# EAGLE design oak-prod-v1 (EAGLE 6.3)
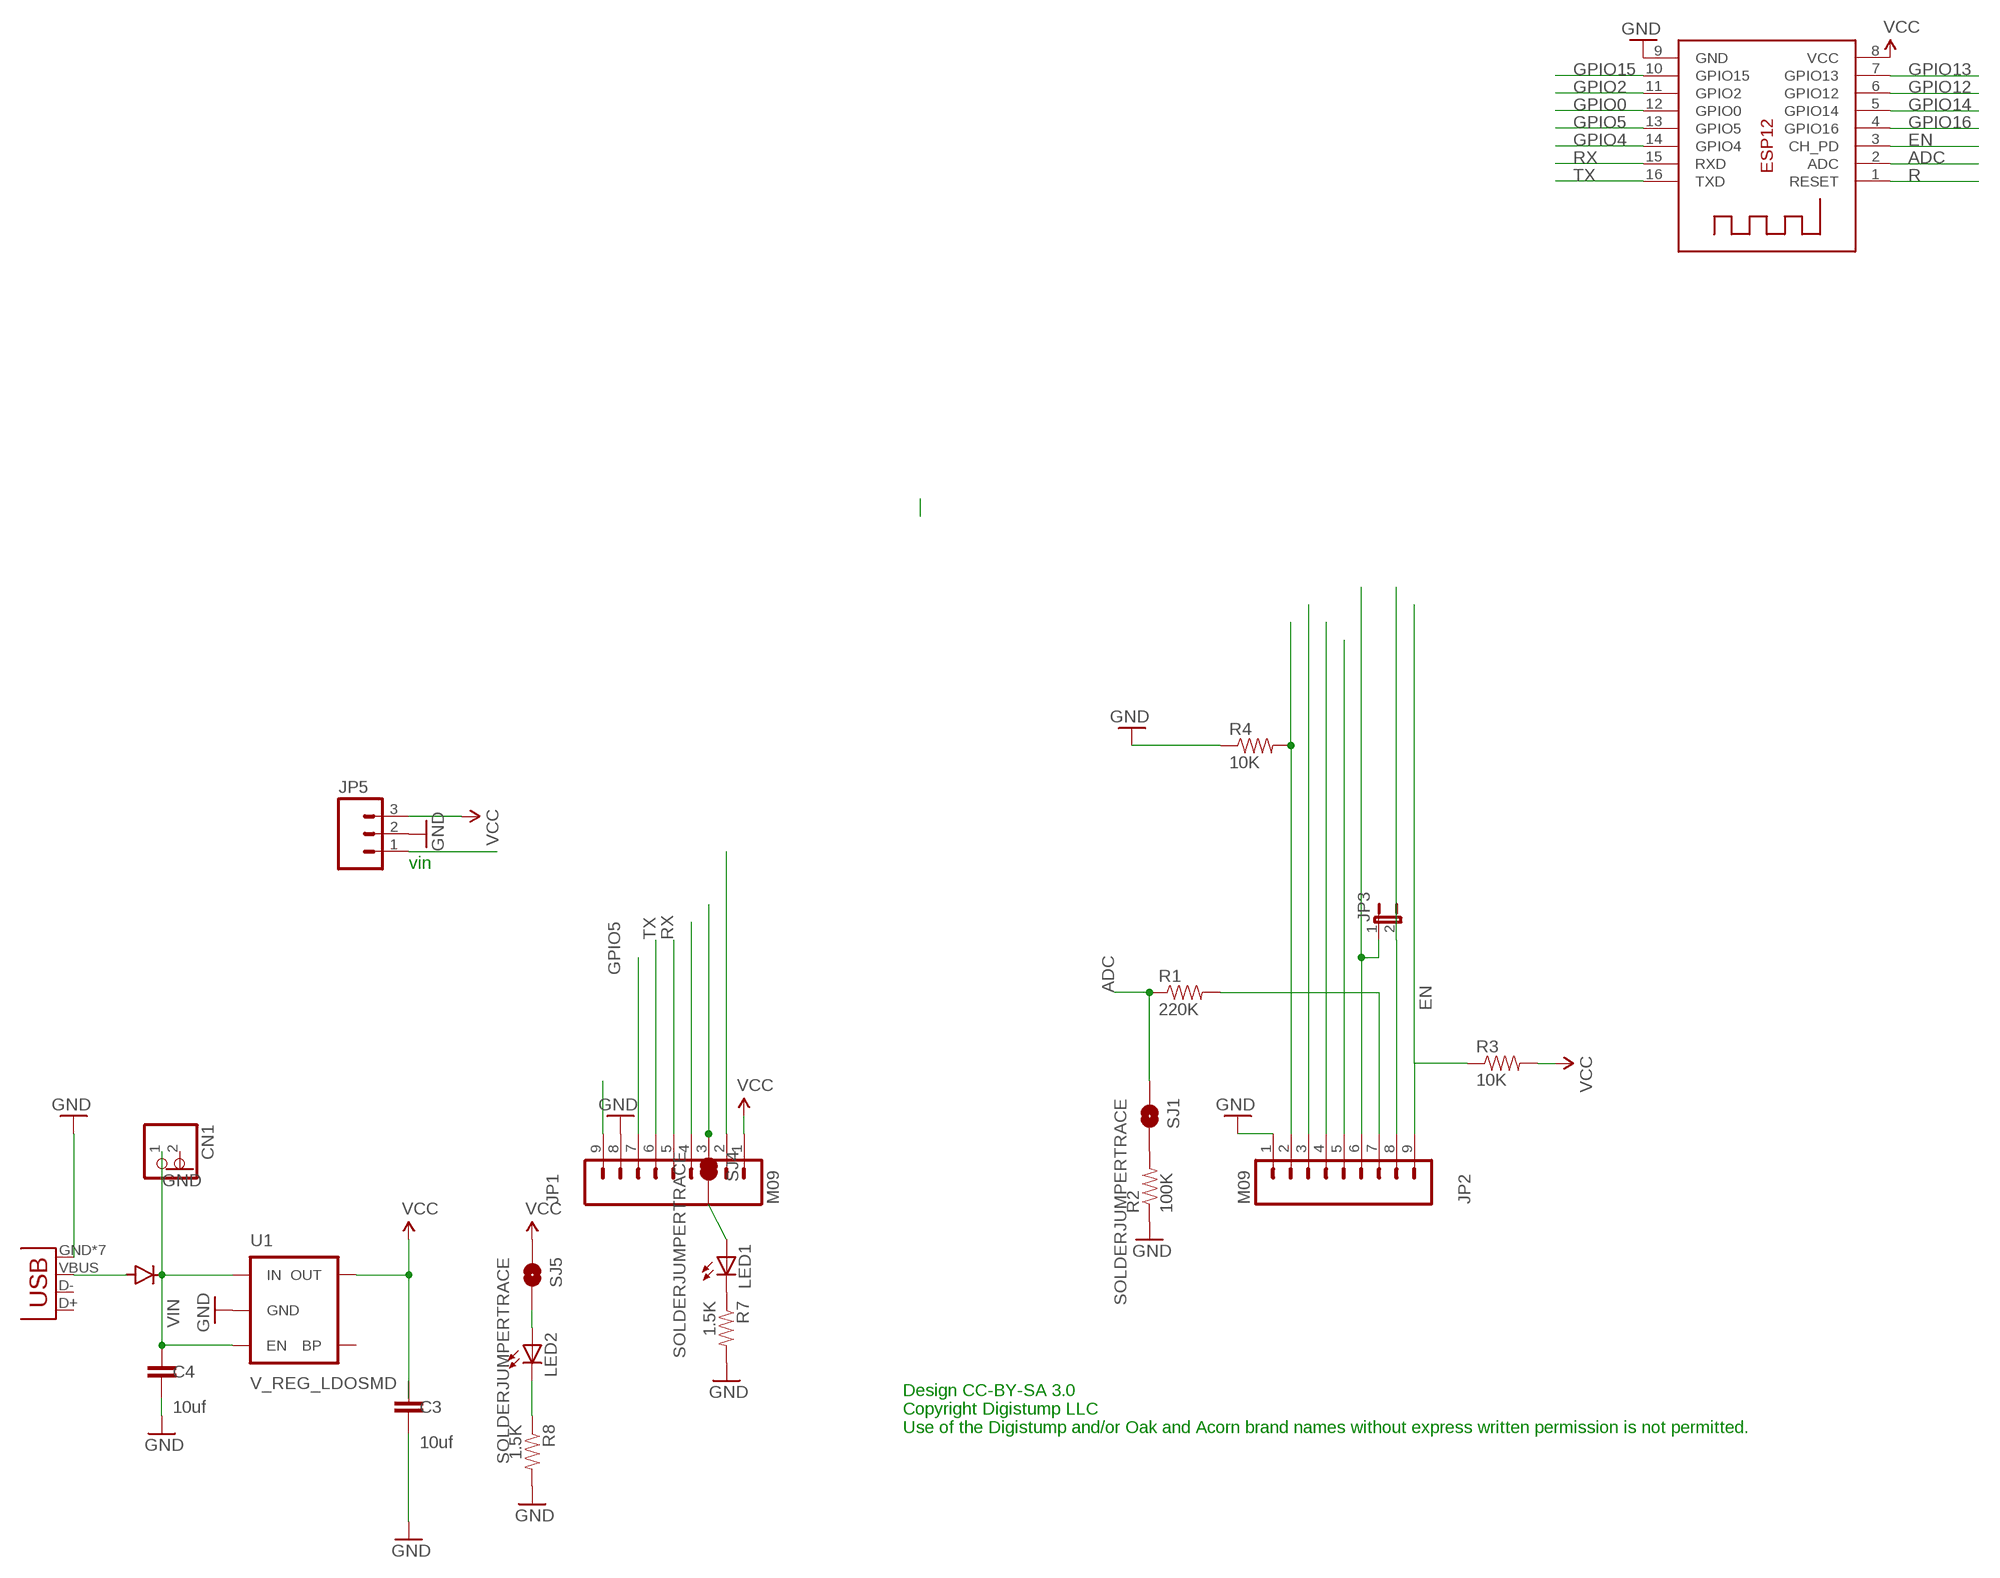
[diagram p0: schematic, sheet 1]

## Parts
C3  10uf  CAP0805  [0805]
C4  10uf  CAP0805  [0805]
CN1  JST_2PIN-THM-RA  [JST-PH-2-THM-RA]
D2  DIODE  [DIODE-DO-220AA(SMP)]
JP1  M09  [1X09]
JP2  M09  [1X09]
JP3  JUMPER-2SMD-NO  [SJ_2S-NO]
JP5  M03PTH  [1X03]
LED1  LEDCHIP-LED0805  [CHIP-LED0805]
LED2  LEDCHIP-LED0805  [CHIP-LED0805]
R1  220K  RESISTOR0603-RES  [0603-RES]
R2  100K  RESISTOR0603-RES  [0603-RES]
R3  10K  RESISTOR0603-RES  [0603-RES]
R4  10K  RESISTOR0603-RES  [0603-RES]
R7  1.5K  RESISTOR0603-RES  [0603-RES]
R8  1.5K  RESISTOR0603-RES  [0603-RES]
SJ1  SOLDERJUMPERTRACE  [SJ_2S-TRACE]
SJ4  SOLDERJUMPERTRACE  [SJ_2S-TRACE]
SJ5  SOLDERJUMPERTRACE  [SJ_2S-TRACE]
U1  V_REG_LDOSMD  [SOT23-5]
X1  ESP-12  [ESP-12]
X2  USB-MICROB  [USB-MICROB]

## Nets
ADC: R1.1 SJ1.1 X1.2(ADC)
EN: JP2.9 R3.1 X1.3(CH_PD)
GND [POWER]: C3.2 C4.2 CN1.2 JP1.8 JP2.1 JP5.2 R2.1 R4.1 R7.2 R8.2 U1.2(GND) X1.9(GND) X2.GND X2.P1(GND) X2.P2(GND) X2.P3(GND) X2.P4(GND) X2.P5(GND) X2.P6(GND)
GPIO0: JP1.4 X1.12(GPIO0)
GPIO2: JP1.2 X1.11(GPIO2)
GPIO4: JP1.3 SJ4.1 X1.14(GPIO4)
GPIO5: JP1.7 X1.13(GPIO5)
GPIO12: JP2.4 X1.6(GPIO12)
GPIO13: JP2.3 X1.7(GPIO13)
GPIO14: JP2.5 X1.5(GPIO14)
GPIO15: JP2.2 R4.2 X1.10(GPIO15)
GPIO16: JP2.6 JP3.1 X1.4(GPIO16)
N$4: D2.ANODE X2.VBUS
N$13: JP2.7 R1.2
N$15: R2.2 SJ1.2
N$21: LED1.C R7.1
N$22: LED1.A SJ4.2
N$23: LED2.A SJ5.2
N$24: LED2.C R8.1
R: JP2.8 JP3.2 X1.1(RESET)
RX: JP1.5 X1.15(RXD)
TX: JP1.6 X1.16(TXD)
VCC [POWER]: C3.1 JP1.1 JP5.3 R3.2 SJ5.1 U1.5(OUT) X1.8(VCC)
VIN: C4.1 CN1.1 D2.CATHODE JP1.9 JP5.1 U1.1(IN) U1.3(EN)
Unconnected: U1.4(BP) X2.D+ X2.D-

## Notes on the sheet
- vin
- Design CC-BY-SA 3.0
  Copyright Digistump LLC
  Use of the Digistump and/or Oak and Acorn brand names without express written permission is not permitted.

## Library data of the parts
C3 C4 = SparkFun-Passives:CAP: Capacitor
CN1 = adafruit:JST_2PIN: JST 2-Pin Connectors of various flavors
D2 = Spark:DIODE
JP1 JP2 = SparkFun:M09: Header 9 Standard 9-pin 0.1" header. Use with straight break away headers (SKU : PRT-00116), right angle break away headers (PRT-00553), swiss pins (PRT-00743), machine pins (PRT-00117), and female headers (PRT-00115).
JP3 = SparkFun:JUMPER-2: Jumper
JP5 = SparkFun:M03: Header 3 Standard 3-pin 0.1" header. Use with straight break away headers (SKU : PRT-00116), right angle break away headers (PRT-00553), swiss pins (PRT-00743), machine pins (PRT-00117), and female headers (PRT-00115). Molex polarized connector foot print use with SKU : PRT-08232 with associated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
LED1 LED2 = adafruit:LED: LED
R1-R4 R7 R8 = SparkFun-Passives:RESISTOR: Resistor
SJ1 SJ4 SJ5 = SparkFun:SOLDERJUMPER: Solder Jumper
U1 = SparkFun:V_REG_LDO: Voltage Regulator LDO Standard 150mA LDO voltage regulator in SOT-23 layout. Micrel part MIC5205. BP (by-pass) pin is used to lower output noise with 470pF cap.
X1 = adafruit:ESP-12
X2 = embeddedmicro:USB: USB Connectors USB-B-PTH is fully proven SKU : PRT-00139/CONN-08278 USB-miniB is fully proven SKU : PRT-00587 USB-A-PCB is untested. USB-A-H is throughly reviewed, but untested. Spark Fun Electronics SKU : PRT-00437 USB-B-SMT is throughly reviewed, but untested. Needs silkscreen touching up.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; PROD_ID: CONN-09505

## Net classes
1 POWER: width 0.203 mm

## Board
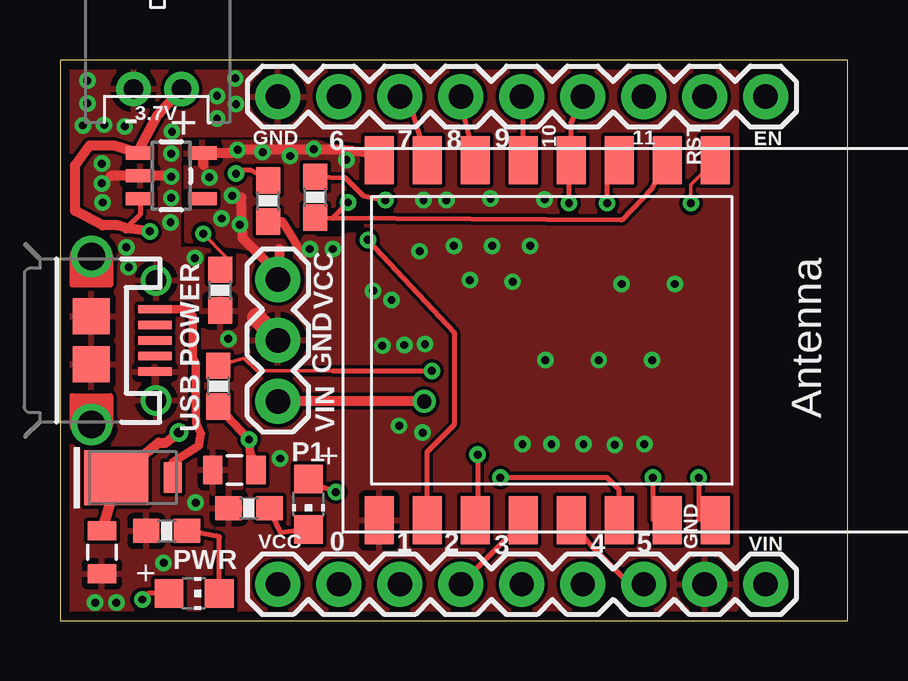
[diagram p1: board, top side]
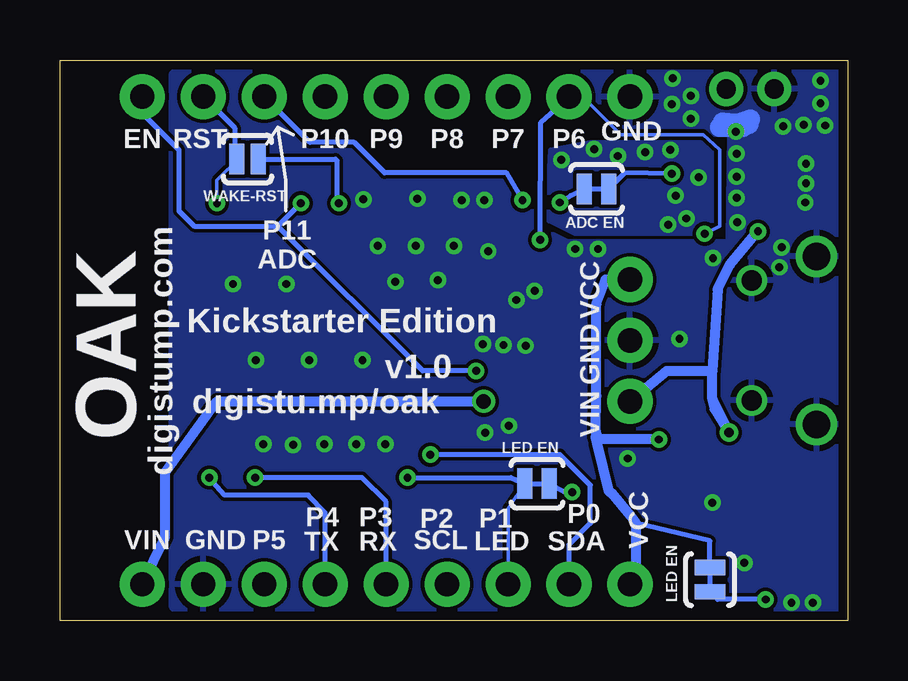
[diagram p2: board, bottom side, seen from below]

Size 32.83 x 23.37 mm. Coordinates in mm from the lower left corner, seen from the top.
Outline: 0,23.37 0,0 32.83,0 32.83,23.37 0,23.37
Copper layers (1*16): Top 0.0356mm / dielectric 1.5011mm / Bottom 0.0356mm
Design rules "default *": minimum track width 6mil, minimum drill 13mil, track to track 6mil, track to pad 8mil, pad to pad 8mil, via to via 8mil, smd to smd 6mil, copper to edge 15mil, drill to drill 8mil, minimum pad ring 7mil, minimum via ring 7mil, stop-mask expansion 4mil, vias tented up to drill 20mil, thermal gap 10mil

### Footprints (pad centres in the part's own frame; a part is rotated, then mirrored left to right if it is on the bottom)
0805 = smd 0.8 x 1.2: 1 -0.9,0; 2 0.9,0
JST-PH-2-THM-RA = drill 0.8 pad 1.422: 1 1,0; 2 -1,0
DIODE-DO-220AA(SMP) = smd 0.762 x 1.27: ANODE 2.349,0 | smd 2.667 x 2.286: CATHODE 0,0
1X09 = drill 1.016 pad 1.88: 1 0,0; 2 2.54,0; 3 5.08,0; 4 7.62,0; 5 10.16,0; 6 12.7,0; 7 15.24,0; 8 17.78,0; 9 20.32,0
SJ_2S-NO = smd 0.635 x 1.27: 1 -0.45,0; 2 0.45,0
1X03 = drill 1.016 pad 1.88: 1 0,0; 2 2.54,0; 3 5.08,0
CHIP-LED0805 = smd 1.2 x 1.2: A 0,-1.05; C 0,1.05
0603-RES = smd 1.1 x 1: 1 -0.85,0; 2 0.85,0
SJ_2S-TRACE = smd 0.635 x 1.27: 1 -0.508,0; 2 0.508,0
SOT23-5 = smd 0.55 x 1.2: 1 -0.95,-1.3; 2 0,-1.3; 3 0.95,-1.3; 4 0.95,1.3; 5 -0.95,1.3
ESP-12 = smd 2 x 1.2: 1 -7.5,4.5; 2 -7.5,2.5; 3 -7.5,0.5; 4 -7.5,-1.5; 5 -7.5,-3.5; 6 -7.5,-5.5; 7 -7.5,-7.5; 8 -7.5,-9.5; 9 7.5,-9.5; 10 7.5,-7.5; 11 7.5,-5.5; 12 7.5,-3.5; 13 7.5,-1.5; 14 7.5,0.5; 15 7.5,2.5; 16 7.5,4.5
USB-MICROB = smd 0.35 x 1.4: D+ 0,2.65; D- -0.65,2.65; GND 1.3,2.65; ID 0.65,2.65; VBUS -1.3,2.65 | smd 1.5 x 1.55: P1 -1,0; P2 1,0 | drill 1.15 pad 1.422: P3 -3.5,0; P4 3.5,0 | drill 0.85 pad 1.27: P5 -2.5,2.7; P6 2.5,2.7

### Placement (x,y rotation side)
C3  7.27,6.29 180 top
C4  1.75,2.86 270 top
CN1  4.06,22.16 0 top
D2  2.35,5.97 0 top
JP1  9.08,1.52 0 top
JP2  9.08,21.84 0 top
JP3  25.02,19.24 180 bottom
JP5  9.08,9.14 90 top
LED1  10.35,4.86 180 top
LED2  5.59,1.14 270 top
R1  10.64,17.65 90 top
R2  8.67,17.49 90 top
R3  6.6,9.78 270 top
R4  6.67,13.78 90 top
R7  7.87,4.7 180 top
R8  4.45,3.75 180 top
SJ1  10.48,18 0 bottom
SJ4  12.95,5.72 0 bottom
SJ5  5.75,1.71 270 bottom
U1  4.64,18.54 270 top
X1  22.8,11.68 270 top
X2  1.31,11.68 270 top

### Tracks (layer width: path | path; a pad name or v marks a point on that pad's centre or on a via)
ADC  (via drill 0.33)
  Top 0.203: X1.2 24.66,17.99 23.4,16.7 10.83,16.76 R1.1 11.37,16.77 v12,17.43
  Bottom 0.203: 10.99,18.03 SJ1.1 11.56,17.72 v12,17.43
EN  (via drill 0.33)
  Top 0.152: R3.1 7.66,10.95 8.19,10.41 11.37,10.41
  Top 0.203: v22.8,17.4 22.8,19.05 X1.3 | 11.37,10.41 v15.49,10.41
  Bottom 0.203: JP2.9 29.4,21.15 27.88,19.62 27.88,17.08 27.24,16.45 23.75,16.45 | 23.75,16.45 v22.8,17.4 | v15.49,10.41 17.72,10.41 23.75,16.45
GND  (via drill 0.33)
  Top 0.356: R2.1 9.26,16.64 9.78,15.81 10.1,15.18
  Top 0.406: v4.64,18.51 4.6,18.54 2.13,18.54
  Top 0.813: JP5.2 9.08,11.75 8.19,12.64
  Bottom 0.813: 5.33,20.57 4.38,20.57 4.06,20.89 4.57,20.73 4.13,20.7 5.21,20.77
  other vias: 1.46,0.76 2.35,0.76 5.65,4.92 4.32,2.41 4.64,17.62 4.64,19.46 1.75,18.22 4.6,16.61 1.14,22.51 1.14,21.56 0.95,20.64 1.84,20.67 2.7,20.61 6.54,20.92 6.54,21.88 10.41,15.49 7.02,11.75 11.37,15.49 20.19,17.56 15.14,17.53 2.86,14.73 9.18,6.76 15.21,11.53 16.1,17.53 17.94,17.59 19.27,7.37 16.41,15.62 18,15.62 19.59,15.62 20.22,10.86 22.45,10.86 24.67,10.86 23.4,14.03 25.62,14.03 21.81,7.37 24.35,7.37 14.13,8.13 15.11,7.84 13.81,13.37 14.35,11.49 13.43,11.46 1.78,17.43 1.75,19.05 7.3,22.61 7.33,21.53 5.62,15.11 2.76,15.56 13.05,13.75 14.99,15.4 17.08,14.19 18.86,14.13 20.48,7.37 23.11,7.33 4.67,20.38
  pour Top: -0.06,23.43 -0.06,16.76 0.25,16.76 0.57,16.45 2.16,16.45 3.68,15.59 4.95,15.53 4.95,15.78 4.98,20.26 11.37,20.26 12.92,19.72 12.89,16.8 12.57,16.07 11.97,16.07 11.81,15.91 10.67,15.91 10.57,16 10.22,16 9.08,13.87 7.68,15.18 5.65,15.49 3.71,15.43 2.16,16.13 0.57,16.13 0.25,16.45 0.25,15.49 -0.06,15.18 -0.06,0.25 0.89,-0.06 27.56,-0.06 28.19,0.57 28.19,22.8 27.56,23.43
  pour Bottom: 27.56,23.43 5.02,23.43 5.02,20.26 11.68,20.26 12.95,19.69 12.95,16.45 11.68,15.81 4.98,15.81 4.89,23.4 -0.06,23.43 -0.06,0.25 0.89,-0.06 27.56,-0.06 28.19,0.57 28.19,22.8
GPIO0
  Top 0.203: X1.12 18.66,3.49 JP1.4
GPIO2  (via drill 0.33)
  Top 0.203: v17.4,6.92 17.4,4.29 X1.11
  Bottom 0.203: JP1.2 11.62,3.18 10.73,4.06 10.73,5.65 12,6.92 16.76,6.92 v17.4,6.92
GPIO4  (via drill 0.33)
  Top 0.203: X1.14 23.3,5.47 22.8,5.97 v18.35,5.97
  Bottom 0.152: JP1.3 14.16,4.7 SJ4.1
  Bottom 0.203: v18.35,5.97 14.03,5.97 SJ4.1
GPIO5
  Top 0.203: JP1.7 23.75,1.52 22.16,3.11 X1.13
GPIO12
  Top 0.203: X1.6 16.66,21.8 JP2.4
GPIO13
  Top 0.203: X1.7 14.66,21.34 JP2.3
GPIO14
  Top 0.203: X1.5 19.3,21.27 JP2.5
GPIO15  (via drill 0.33)
  Top 0.152: R4.2 6.91,15.17 v5.97,16.13
  Top 0.203: X1.10 15.3,7.04 16.45,8.19 16.45,12 v12.83,15.88
  Bottom 0.152: v5.97,16.13 5.33,16.45 5.33,19.62 6.03,20.26 9.46,20.26 11.05,21.84 JP2.2
  Bottom 0.203: v12.83,15.88 12.8,20.77 JP2.2
GPIO16  (via drill 0.33)
  Top 0.203: JP2.6 21.3,20.73 X1.4 21.21,19.1 v21.21,17.4
  Bottom 0.152: JP3.1 24.57,19.37
  Bottom 0.203: JP3.1 21.35,19.24 X1.4 21.3,17.49 v21.21,17.4
N$4
  Top 0.356: D2.ANODE 4.7,6.6 5.78,7.3 5.87,7.81 5.68,8.22 5.65,8.67 5.65,10.73 5.52,10.95 5.52,12.67 5.33,12.95 5.3,12.98 X2.VBUS
N$13  (via drill 0.33)
  Top 0.203: R1.2 11.88,18.47 12.64,17.72 v13.56,17.53
  Bottom 0.203: JP2.7 22.42,19.94 20.57,19.94 19.3,18.67 14.22,18.67 v13.56,17.53
N$15  (via drill 0.33)
  Top 0.203: R2.2 7.97,18.76 7.65,18.76 v7.33,18.64
  Bottom 0.203: 10.1,18.23 SJ1.2 9.3,18.67 v7.33,18.64
N$21
  Top 0.203: LED1.C 9.21,3.67 R7.1
N$22  (via drill 0.33)
  Top 0.203: v11.49,5.37 10.73,5.65 LED1.A
  Bottom 0.203: SJ4.2 11.75,5.33 v11.49,5.37
N$23  (via drill 0.33)
  Top 0.203: LED2.A 3.68,1.14 v3.43,0.89
  Bottom 0.203: v3.43,0.89 5.43,0.89 SJ5.2
N$24
  Top 0.203: LED2.C 6.64,3.5 R8.1
R  (via drill 0.33)
  Top 0.152: v26.29,17.4 26.29,18.18 X1.1
  Bottom 0.152: JP3.2 25.53,19.3 25.34,19.3 26.29,18.35 v26.29,17.4
  Bottom 0.203: 25.53,19.3 25.53,20.52 JP2.8
RX  (via drill 0.33)
  Top 0.203: v24.7,5.97 24.7,4.22 X1.15
  Bottom 0.203: JP1.5 19.24,4.95 20.26,5.97 v24.7,5.97
TX  (via drill 0.33)
  Top 0.203: v26.61,5.97 26.61,4.24 X1.16
  Bottom 0.203: JP1.6 21.78,4.51 22.48,5.24 25.97,5.24 v26.61,5.97
VCC  (via drill 0.33)
  Top 0.356: R3.2 v7.87,7.56 7.92,6.97 C3.1
  Top 0.406: JP5.3 8.83,14.73 7.62,15.94 7.56,17.63 | X1.8 12.79,19.5 11.68,19.62 v7.4,19.62 | 9.14,15.49 9.14,14.22 | 5.97,19.3 5.97,18.99 5.97,19.46 6,19.49 7.18,19.49
  Bottom 0.203: SJ5.1 5.75,3.33 8.83,4.06
  Bottom 0.406: JP1.1 8.83,1.52 8.83,4.06 9.05,4.38 9.84,5.33 9.94,5.37 10.45,7.4 10.52,7.66 10.41,7.56 | v7.87,7.56 10.41,7.56 | 10.41,7.56 10.51,7.97 10.48,9.37 10.48,13.21 10.1,14.22 JP5.3
  other vias: 6.22,18.48 7.18,17.72 6.73,16.76 7.49,16.51 9.59,19.37 10.57,19.65 8.45,19.53 11.94,19.21
  pour Bottom: 5.24,19.94 5.24,16.13 11.37,16.13 12.45,16.67 12.41,18.86 12.38,19.62 10.73,19.94
  pour Top: 5.24,19.94 5.27,15.84 5.94,15.78 7.59,15.59 9.43,15.24 9.59,16.35 11.18,16.54 12.48,16.73 12.41,19.37 10.73,19.94
VIN  (via drill 0.33, 0.41, 0.6)
  Top 0.203: 0.57,17.59 0.63,17.4 | U1.3 3.34,16.93 2.76,16.35
  Top 0.406: C4.1 2.06,4.79 D2.CATHODE 4.1,7.43 4.41,7.43 v4.95,7.84 | v3.75,16.22 2.76,16.35 2.42,16.48 1.78,16.48 0.63,17.08 0.63,17.4 0.63,18.99 1.24,19.81 2.25,19.81 U1.1 3.3,19.65 4.06,21.08 5.02,22.11 CN1.1 | v15.18,9.14 JP5.1
  Bottom 0.406: JP1.9 28.45,3.49 28.45,6.19 26.29,9.14 v15.18,9.14 | JP5.1 7.56,10.41 5.65,10.41 | 5.65,9.24 5.56,8.83 v4.95,7.84 5.65,9.24 | v3.75,16.22 4.92,14.83 5.43,13.81 5.65,10.41 | 5.65,9.24 5.65,10.41

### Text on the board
tPlace: 3.7V | GND | 6 | 7 | 8 | 9 | 10 | 11 | EN | RST | USB POWER | VCC | GND | P1 | VIN | VCC | 3 | VIN | 0 | 1 | 2 | 4 | 5 | GND | PWR
bPlace: GND | P6 | P7 | P8 | P9 | P10 | RST | EN | WAKE-RST | P11 / ADC | ADC EN | digistump.com | OAK | VCC | GND | Kickstarter Edition | VIN | v1.0 | digistu.mp/oak | LED EN | VCC | P0 | P1 | SDA | LED | P2 | P3 | P4 | LED EN | SCL | RX | TX | P5 | GND | VIN
bOrigins: MOSI | MISO | SCK | WAKE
